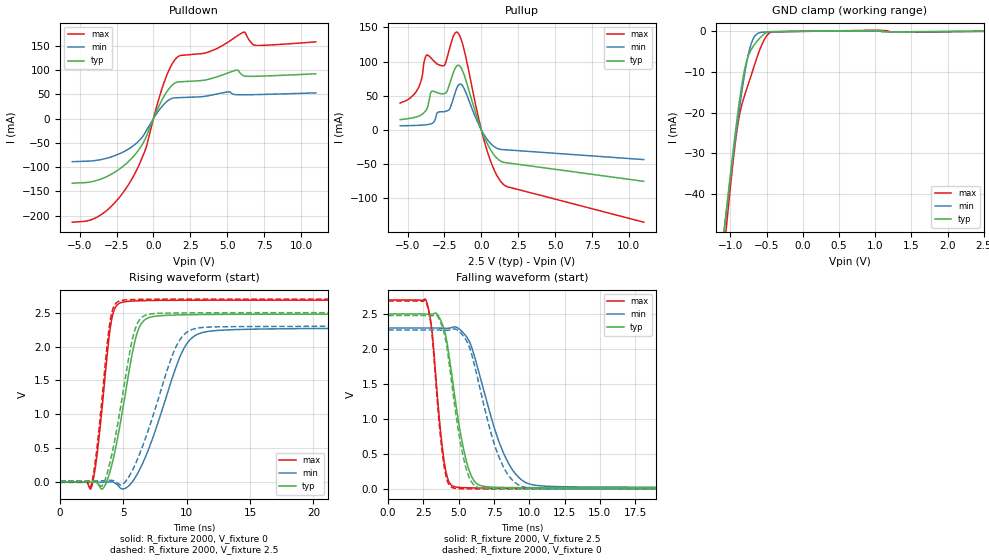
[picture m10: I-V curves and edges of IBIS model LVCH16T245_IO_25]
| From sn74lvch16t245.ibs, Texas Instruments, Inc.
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[Model]   LVCH16T245_IO_25
Model_type  I/O
Vinl=0.7
Vinh=1.7
Enable   Active-Low
Vref =   0
Rref =   2000
Cref =   15p
Vmeas =   1.25
| variable   typ   min   max
C_comp   6.25pF   5.27pF   7.45pF
| C_pullup   12.85pF   6.61pF   21.54pF
| C_pulldown   9.85pF   6.67pF   15.53pF
| C_tri-state   6.25pF   5.27pF   7.45pF
[Temperature Range]   40   100   -40
| Ambient temperature   25   85   -40
[Voltage range]   2.5   2.3   2.7
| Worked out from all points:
|   slope of the pulldown table from 0 to 0.375 V, typ, clamps not added: 14.3 ohm
|   slope of the pullup table from 0 to 0.375 V, typ, clamps not added: 19.7 ohm
|   GND clamp passes 1 mA (typ) near -0.56 V on its own axis
|   rising waveform, R_fixture 2000, V_fixture 0: 20-80 % time 1.41ns typ, 2.48ns min, 873ps max; typ from 0 V to 2.48 V
|   falling waveform, R_fixture 2000, V_fixture 2.5: 20-80 % time 1.17ns typ, 2.07ns min, 714ps max; typ from 2.5 V to 0.017 V
|   rising waveform, R_fixture 2000, V_fixture 2.5: 20-80 % time 1.39ns typ, 2.41ns min, 860ps max; typ from 0.017 V to 2.5 V
|   falling waveform, R_fixture 2000, V_fixture 0: 20-80 % time 1.09ns typ, 1.8ns min, 688ps max; typ from 2.48 V to 0 V
[GND Clamp]
| LVCH16T245_IO_25
|   Voltage   I(typ)   I(min)   I(max)
-5.5V     -898.4mA   -832.8mA   -1.017A
-1.085V   -48.77mA   -48.67mA   -53.42mA
-1.055V   -43.87mA   -44.14mA   -47.92mA
-960mV    -28.98mA   -30.27mA   -31.59mA
-900mV    -20.36mA   -22.06mA   -23.19mA
-845mV    -13.46mA   -15.11mA   -18.23mA
-785mV    -7.911mA   -8.547mA   -14.72mA
-730mV    -5.074mA   -4.049mA   -11.75mA
-665mV    -3.171mA   -1.227mA   -8.154mA
-555mV    -972.5uA   -214.6uA   -2.841mA
-465mV    -115.2uA   -117.2uA   -458.8uA
2.5V      30.12pA    299.1nA    -54.31nA
[Pulldown]
| LVCH16T245_IO_25
|   Voltage   I(typ)   I(min)   I(max)
-5.5V     -133.3mA   -88.88mA   -213.8mA
-3.55V    -124.7mA   -84.51mA   -198.3mA
-1.715V   -89.25mA   -63.13mA   -137.4mA
-555mV    -41.71mA   -28.61mA   -64.74mA
300mV     21.24mA    14.01mA    33.98mA
855mV     53.14mA    33.96mA    85.74mA
1.655V    75.71mA    43.25mA    127.8mA
3.765V    81.48mA    47.49mA    138mA
5.655V    100.3mA    49.41mA    170.3mA
6.145V    88.26mA    49.23mA    178.7mA
6.91V     87.46mA    49.58mA    151.3mA
11V       92.57mA    53.16mA    158.4mA
[Pullup]
| LVCH16T245_IO_25
|   Voltage   I(typ)   I(min)   I(max)
-5.5V     15.18mA    6.286mA    39.52mA
-4.375V   19.38mA    6.776mA    57.63mA
-3.925V   24.63mA    7.34mA     94.35mA
-3.695V   31.09mA    7.844mA    109.8mA
-3.295V   56.83mA    10.28mA    102.6mA
-2.495V   53.5mA     27.01mA    94.85mA
-2.135V   68.6mA     31.44mA    120.9mA
-1.645V   94.12mA    62.3mA     143.1mA
-1.23V    84.36mA    63.07mA    122.5mA
335mV     -17.24mA   -11.96mA   -26.61mA
1.44V     -46.81mA   -28.58mA   -78.45mA
11V       -75.01mA   -43.22mA   -134.8mA
[Ramp]
| LVCH16T245_IO_25
| variable   typ   min   max
dV/dt_r   1.54/1.48E-09   1.42/2.61E-09   1.67/9.11E-10
dV/dt_f   1.50/1.18E-09   1.38/2.08E-09   1.62/7.19E-10
R_load = 2000
[Rising Waveform]
| LVCH16T245_IO_25
R_fixture =   2000
C_fixture =   0
L_fixture =   0
V_fixture =   0
V_fixture_min = 0
V_fixture_max = 0
|   Time   V(typ)   V(min)   V(max)
0s        330.6pV    7.312nV    2.064nV
2.475ns   -49.77uV   -5.235uV   -70.2mV
2.97ns    -22.42mV   -29.92uV   493.8mV
4.005ns   204.2mV    6.57mV     2.332V
4.79ns    912.3mV    -91.16mV   2.647V
5.815ns   2.01V      37.41mV    2.671V
6.46ns    2.351V     257.2mV    2.676V
9.52ns    2.467V     1.875V     2.683V
11.02ns   2.472V     2.194V     2.683V
40ns      2.477V     2.27V      2.684V
[Falling Waveform]
| LVCH16T245_IO_25
R_fixture =   2000
C_fixture =   0
L_fixture =   0
V_fixture =   2.5
V_fixture_min = 2.3
V_fixture_max = 2.7
|   Time   V(typ)   V(min)   V(max)
0s        2.5V       2.3V       2.7V
2.72ns    2.499V     2.3V       2.679V
3.1ns     2.497V     2.3V       2.277V
3.965ns   2.282V     2.296V     407.2mV
4.66ns    1.416V     2.316V     37.39mV
5.415ns   511.3mV    2.21V      20.81mV
6.11ns    113.7mV    1.901V     17.62mV
8.12ns    24.8mV     541mV      14.09mV
9.99ns    21.71mV    75.12mV    12.91mV
40ns      16.63mV    23.17mV    11.24mV
[Rising Waveform]
| LVCH16T245_IO_25
R_fixture =   2000
C_fixture =   0
L_fixture =   0
V_fixture =   2.5
V_fixture_min = 2.3
V_fixture_max = 2.7
|   Time   V(typ)   V(min)   V(max)
0s        16.56mV    22.85mV    11.23mV
2.425ns   16.42mV    22.85mV    -58.3mV
3.3ns     -54.38mV   22.73mV    1.221V
3.925ns   286mV      27.93mV    2.352V
4.675ns   999.5mV    -31.23mV   2.672V
5.635ns   2.051V     151.2mV    2.692V
6.26ns    2.392V     410.6mV    2.695V
8.995ns   2.494V     1.935V     2.699V
10.44ns   2.497V     2.252V     2.7V
40ns      2.5V       2.3V       2.7V
[Falling Waveform]
| LVCH16T245_IO_25
R_fixture =   2000
C_fixture =   0
L_fixture =   0
V_fixture =   0
V_fixture_min = 0
V_fixture_max = 0
|   Time   V(typ)   V(min)   V(max)
0s        2.478V     2.272V     2.685V
2.715ns   2.477V     2.272V     2.664V
3.085ns   2.475V     2.272V     2.26V
3.925ns   2.263V     2.268V     384.9mV
4.58ns    1.405V     2.283V     19.95mV
5.285ns   497.6mV    2.196V     5.473mV
5.955ns   89.72mV    1.901V     3.771mV
7.785ns   3.178mV    493.3mV    1.904mV
9.53ns    2.444mV    34.47mV    1.234mV
40ns      55.77uV    202.1uV    6.683uV
